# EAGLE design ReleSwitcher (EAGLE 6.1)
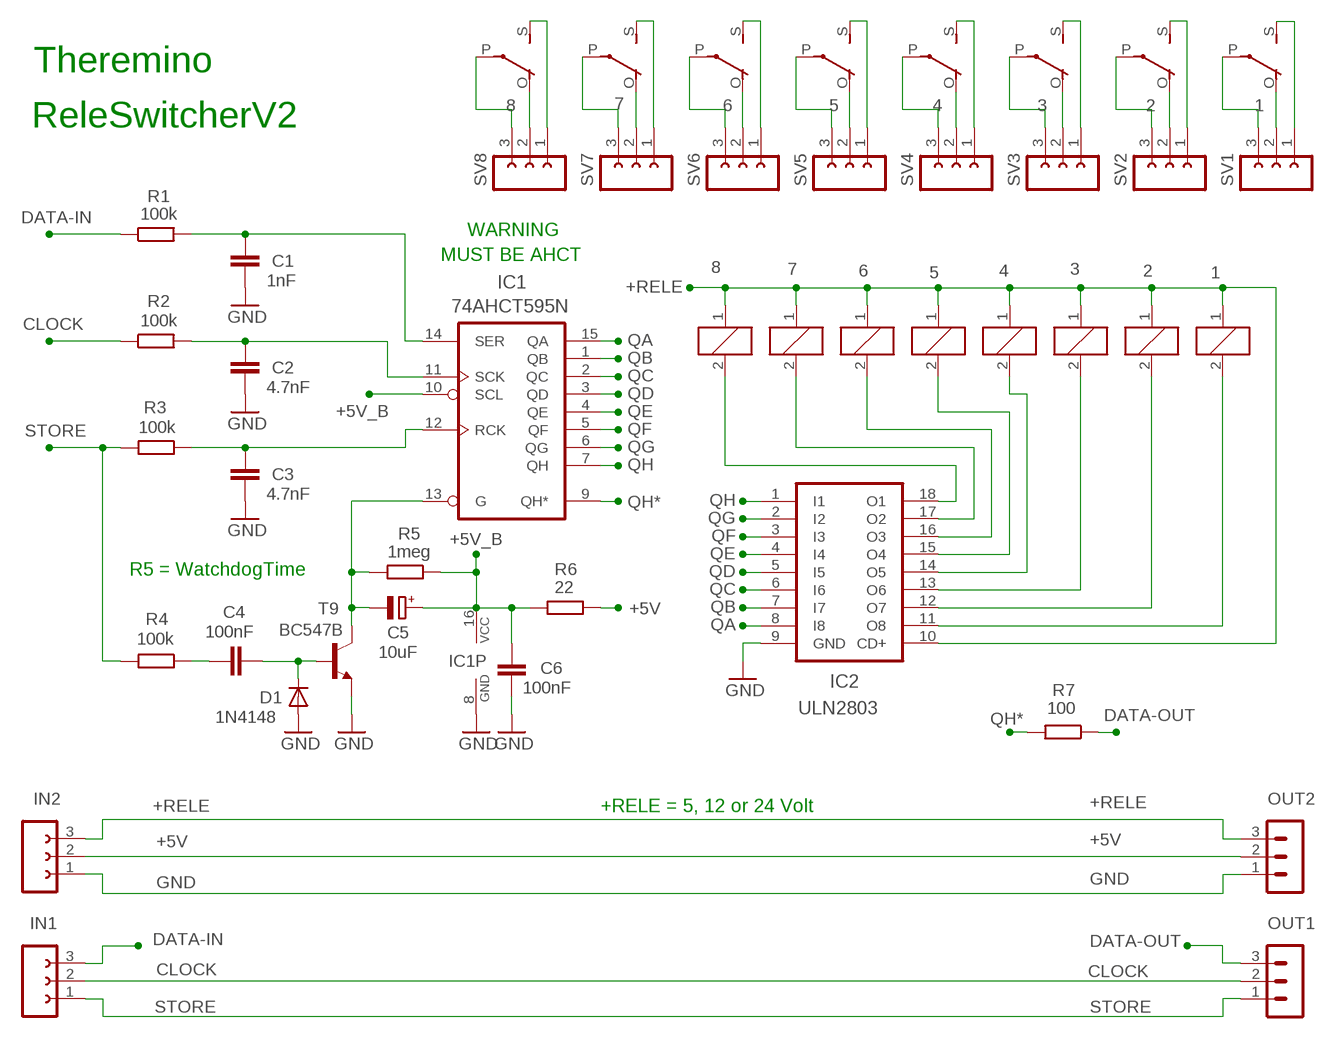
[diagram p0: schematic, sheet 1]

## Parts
1  E3206S  [E3206S]
2  E3206S  [E3206S]
3  E3206S  [E3206S]
4  E3206S  [E3206S]
5  E3206S  [E3206S]
6  E3206S  [E3206S]
7  E3206S  [E3206S]
8  E3206S  [E3206S]
C1  1nF  C-EU025-024X044  [C025-024X044]
C2  4.7nF  C-EU025-024X044  [C025-024X044]
C3  4.7nF  C-EU025-024X044  [C025-024X044]
C4  100nF  C-EU025-024X044  [C025-024X044]
C5  10uF  CPOL-EUE15-5AXIAL  [E15-5]
C6  100nF  C-EU025-024X044  [C025-024X044]
D1  1N4148  DIODE-D-5  [D-5]
IC1  74AHCT595N  74HCT595N  [DIL16]
IC2  ULN2803  ULN2803A  [DIL18]
IN1  FE03-1"  [FE03-1]
IN2  FE03-1"  [FE03-1]
OUT1  MA03-1N  [MA03-1]
OUT2  MA03-1N  [MA03-1]
R1  100k  R-EU_0207/10  [0207/10]
R2  100k  R-EU_0207/10  [0207/10]
R3  100k  R-EU_0207/10  [0207/10]
R4  100k  R-EU_0207/10  [0207/10]
R5  1meg  R-EU_0207/10  [0207/10]
R6  22  R-EU_0207/10  [0207/10]
R7  100  R-EU_0207/10  [0207/10]
SV1  CN-03"  [CN-03]
SV2  CN-03"  [CN-03]
SV3  CN-03"  [CN-03]
SV4  CN-03"  [CN-03]
SV5  CN-03"  [CN-03]
SV6  CN-03"  [CN-03]
SV7  CN-03"  [CN-03]
SV8  CN-03"  [CN-03]
T9  BC547B  -NPN-TO92-CBE  [TO92-CBE]

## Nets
+5V: IN2.2 OUT2.2 R6.1
+5V_B: C5.+ C6.1 IC1.10(SCL) IC1.16(VCC) R5.1 R6.2
+RELE: 1.1 2.1 3.1 4.1 5.1 6.1 7.1 8.1 IC2.10(CD+) IN2.3 OUT2.3
CLOCK: IN1.2 OUT1.2 R2.1
DATA-IN: IN1.3 R1.1
DATA-OUT: OUT1.3 R7.1
GND: C1.2 C2.2 C3.2 C6.2 D1.A IC1.8(GND) IC2.9(GND) IN2.1 OUT2.1 T9.E
N$1: 1.O(2:O) SV1.2
N$2: 1.P(2:P) SV1.3
N$3: C2.1 IC1.11(SCK) R2.2
N$4: 1.S(2:S) SV1.1
N$5: 2.S(2:S) SV2.1
N$6: 2.O(2:O) SV2.2
N$7: 3.2 IC2.13(O6)
N$8: 2.P(2:P) SV2.3
N$9: 3.S(2:S) SV3.1
N$10: 5.2 IC2.15(O4)
N$11: 6.2 IC2.16(O3)
N$12: 7.2 IC2.17(O2)
N$13: 8.2 IC2.18(O1)
N$14: 3.O(2:O) SV3.2
N$15: 3.P(2:P) SV3.3
N$16: C3.1 IC1.12(RCK) R3.1
N$17: C1.1 IC1.14(SER) R1.2
N$18: 4.S(2:S) SV4.1
N$19: 4.O(2:O) SV4.2
N$20: 4.P(2:P) SV4.3
N$21: 5.S(2:S) SV5.1
N$22: 5.O(2:O) SV5.2
N$23: 5.P(2:P) SV5.3
N$24: 6.S(2:S) SV6.1
N$25: 6.O(2:O) SV6.2
N$26: 6.P(2:P) SV6.3
N$27: 1.2 IC2.11(O8)
N$28: 2.2 IC2.12(O7)
N$29: 7.S(2:S) SV7.1
N$30: 4.2 IC2.14(O5)
N$31: 7.O(2:O) SV7.2
N$32: 7.P(2:P) SV7.3
N$33: 8.S(2:S) SV8.1
N$34: 8.O(2:O) SV8.2
N$35: 8.P(2:P) SV8.3
N$36: C4.1 R4.1
N$37: C5.- IC1.13(G) R5.2 T9.C
N$39: C4.2 D1.C T9.B
QA: IC1.15(QA) IC2.8(I8)
QB: IC1.1(QB) IC2.7(I7)
QC: IC1.2(QC) IC2.6(I6)
QD: IC1.3(QD) IC2.5(I5)
QE: IC1.4(QE) IC2.4(I4)
QF: IC1.5(QF) IC2.3(I3)
QG: IC1.6(QG) IC2.2(I2)
QH: IC1.7(QH) IC2.1(I1)
QH*: IC1.9(QH*) R7.2
STORE: IN1.1 OUT1.1 R3.2 R4.2

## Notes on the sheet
- Theremino
- ReleSwitcherV2
- WARNING
- MUST BE AHCT
- R5 = WatchdogTime
- +RELE = 5, 12 or 24 Volt

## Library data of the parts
1-8 = relay:E3206S: RELAY 1 x switch, Eichhoff/distributor Schukat
C1-C4 C6 = 00-LIVIO:C-EU: CAPACITOR, European symbol
C5 = 00-LIVIO:CPOL-EU: POLARIZED CAPACITOR, European symbol
D1 = 00-LIVIO:DIODE-: DIODE
IC1 = 74xx-eu:74*595: 8-bit SHIFT REGISTER, output latch
IC2 = uln-udn:ULN2803A: DRIVER ARRAY
IN1 IN2 = 02-con-lsta-F:FE03-1: FEMALE HEADER
OUT1 OUT2 = 03-con-lstb-M:MA03-1: PIN HEADER
R1-R7 = 00-LIVIO:R-EU_: RESISTOR, European symbol
SV1-SV8 = 01-Connettori_Vite_2.54:CN-03: Screw connector - Green - Spacing 2.54
T9 = 00-LIVIO:*-NPN-: NPN Transistror

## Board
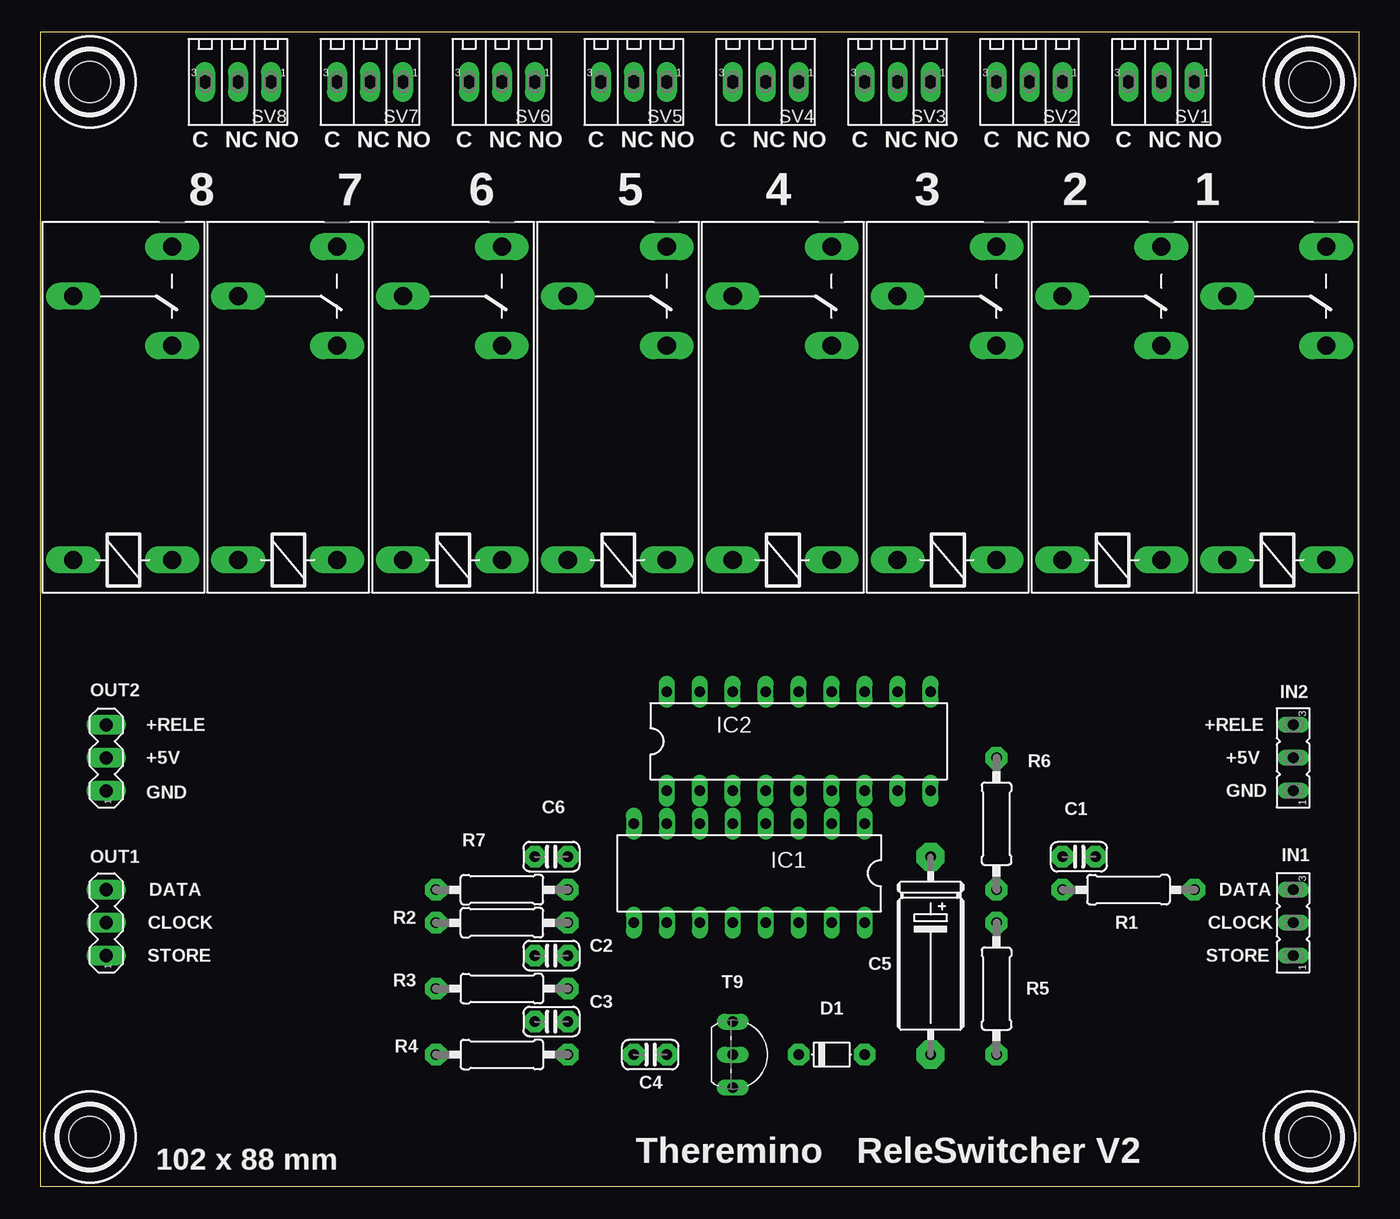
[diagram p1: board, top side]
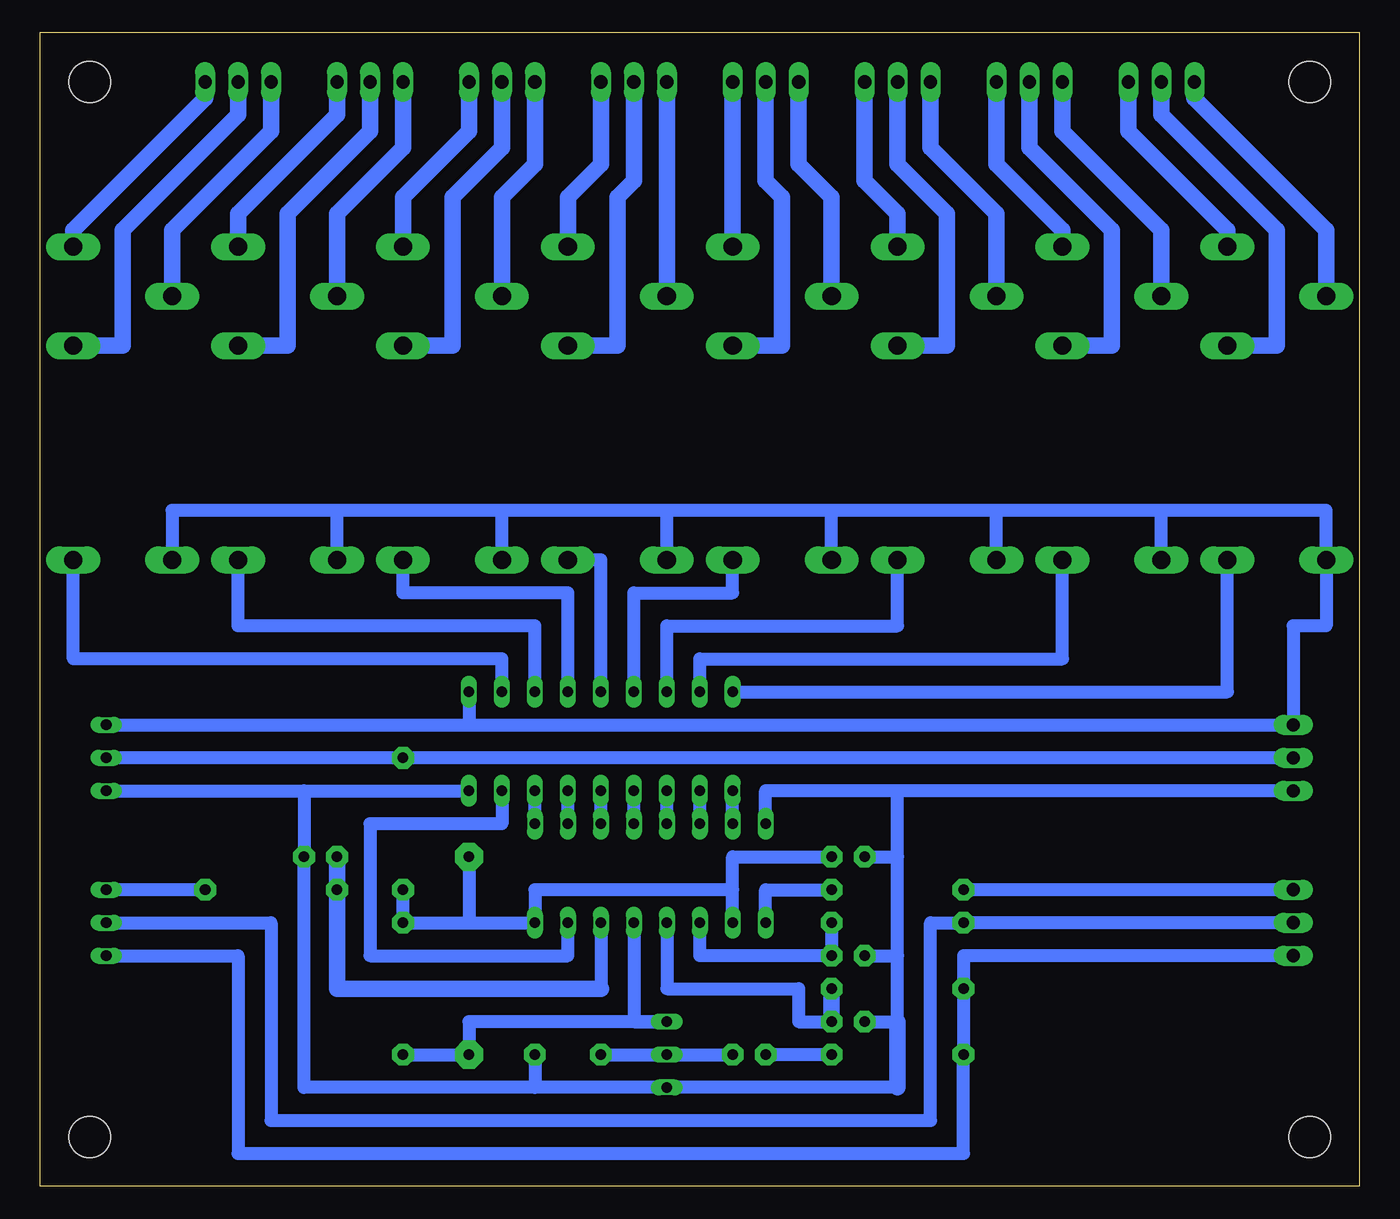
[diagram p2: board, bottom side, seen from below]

Size 101.6 x 88.9 mm. Coordinates in mm from the lower left corner, seen from the top.
Outline: 101.6,88.9 0,88.9 0,0 101.6,0 101.6,88.9
Copper layers (1*16): Top 0.035mm / dielectric 1.5mm / Bottom 0.035mm
Design rules: minimum track width 10mil, minimum drill 31mil, track to track 31mil, track to pad 31mil, pad to pad 31mil, via to via 31mil, smd to smd 31mil, copper to edge 31mil, drill to drill 8mil, minimum pad ring 5mil, minimum via ring 8mil, stop-mask expansion 4mil, vias tented up to drill 0mil, thermal gap 47mil
Holes 3.2 mm at 97.79,85.09 3.81,85.09 3.81,3.81 97.79,3.81

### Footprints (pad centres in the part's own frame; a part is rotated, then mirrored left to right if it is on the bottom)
E3206S = drill 1.397 long: 1 -3.175,3.81; 2 -3.175,-3.81; O 13.335,-3.81; P 17.145,3.81; S 20.955,-3.81
C025-024X044 = drill 0.813 pad 1.676 octagon: 1 -1.27,0; 2 1.27,0
E15-5 = drill 0.813 pad 2.159 octagon: + -7.62,0; - 7.62,0
D-5 = drill 0.813 pad 1.676 octagon: A 2.54,0; C -2.54,0
DIL16 = drill 0.813 long: 1 -8.89,-3.81; 2 -6.35,-3.81; 3 -3.81,-3.81; 4 -1.27,-3.81; 5 1.27,-3.81; 6 3.81,-3.81; 7 6.35,-3.81; 8 8.89,-3.81; 9 8.89,3.81; 10 6.35,3.81; 11 3.81,3.81; 12 1.27,3.81; 13 -1.27,3.81; 14 -3.81,3.81; 15 -6.35,3.81; 16 -8.89,3.81
DIL18 = drill 0.813 long: 1 -10.16,-3.81; 2 -7.62,-3.81; 3 -5.08,-3.81; 4 -2.54,-3.81; 5 0,-3.81; 6 2.54,-3.81; 7 5.08,-3.81; 8 7.62,-3.81; 9 10.16,-3.81; 10 10.16,3.81; 11 7.62,3.81; 12 5.08,3.81; 13 2.54,3.81; 14 0,3.81; 15 -2.54,3.81; 16 -5.08,3.81; 17 -7.62,3.81; 18 -10.16,3.81
FE03-1 = drill 0.813 long: 1 -2.54,0; 2 0,0; 3 2.54,0
MA03-1 = drill 1.016 long: 1 -2.54,0; 2 0,0; 3 2.54,0
0207/10 = drill 0.813 pad 1.676 octagon: 1 -5.08,0; 2 5.08,0
CN-03 = drill 1.016 pad 1.422 long: 1 -2.54,0; 2 0,0; 3 2.54,0
TO92-CBE = drill 0.813 long: B 0,0; C -2.54,0; E 2.54,0

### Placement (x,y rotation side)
1  95.25,51.43 90 top
2  82.55,51.43 90 top
3  69.85,51.43 90 top
4  57.15,51.43 90 top
5  44.45,51.43 90 top
6  31.75,51.43 90 top
7  19.05,51.43 90 top
8  6.35,51.43 90 top
C1  80.01,25.4 0 top
C2  39.37,17.78 180 top
C3  39.37,12.7 180 top
C4  46.99,10.16 0 top
C5  68.58,17.78 270 top
C6  39.37,25.4 180 top
D1  60.96,10.16 0 top
IC1  54.61,24.13 180 top
IC2  58.42,34.29 0 top
IN1  96.52,20.32 90 top
IN2  96.52,33.02 90 top
OUT1  5.08,20.32 90 top
OUT2  5.08,33.02 90 top
R1  83.82,22.86 180 top
R2  35.56,20.32 0 top
R3  35.56,15.24 180 top
R4  35.56,10.16 180 top
R5  73.66,15.24 270 top
R6  73.66,27.94 270 top
R7  35.56,22.86 0 top
SV1  86.36,85.09 180 top
SV2  76.2,85.09 180 top
SV3  66.04,85.09 180 top
SV4  55.88,85.09 180 top
SV5  45.72,85.09 180 top
SV6  35.56,85.09 180 top
SV7  25.4,85.09 180 top
SV8  15.24,85.09 180 top
T9  53.34,10.16 270 top

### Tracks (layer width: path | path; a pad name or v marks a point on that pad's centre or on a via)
+5V
  Bottom 1.016: IN2.2 R6.1 OUT2.2
+5V_B
  Bottom 1.016: 68.58,20.32 R5.1 R6.2 | C5.+ 68.58,20.32 | 68.58,20.32 IC1.16 63.5,22.86 48.26,22.86 IC1.10 48.26,25.4 C6.1
+RELE
  Bottom 1.016: 15.24,52.07 2.54,52.07 8.1 2.54,43.18 5.08,43.18 OUT2.3 68.58,35.56 | 15.24,52.07 27.94,52.07 | 27.94,52.07 40.64,52.07 | 40.64,52.07 53.34,52.07 | 53.34,52.07 66.04,52.07 | 66.04,52.07 78.74,52.07 | 78.74,52.07 91.44,52.07 1.1 | 7.1 15.24,52.07 | 6.1 27.94,52.07 | 5.1 40.64,52.07 | 4.1 53.34,52.07 | 3.1 66.04,52.07 | 2.1 78.74,52.07 | IC2.10 68.58,35.56 | IN2.3 68.58,35.56
CLOCK
  Bottom 1.016: OUT1.2 R2.1 33.02,20.32 33.02,5.08 83.82,5.08 83.82,20.32 IN1.2
DATA-IN
  Bottom 1.016: R1.1 IN1.3
DATA-OUT
  Bottom 1.016: OUT1.3 R7.1
GND
  Bottom 1.016: OUT2.1 35.56,30.48 | 35.56,30.48 45.72,30.48 IC1.8 | 81.28,30.48 IC2.9 | 35.56,7.62 T9.E 63.5,7.62 | 63.5,7.62 81.28,7.62 C1.2 81.28,30.48 | IN2.1 81.28,30.48 | 35.56,17.78 35.56,12.7 C3.2 | 35.56,17.78 35.56,25.4 | 35.56,25.4 35.56,30.48 | C2.2 35.56,17.78 | D1.A 63.5,7.62 | C6.2 35.56,25.4
  Bottom 1.27: 35.56,7.62 35.56,12.7
N$1
  Bottom 1.27: 1.O 95.25,64.77 95.25,73.66 86.36,82.55 SV1.2
N$2
  Bottom 1.27: 1.P 91.44,73.66 83.82,81.28 SV1.3
N$3
  Bottom 1.016: R2.2 C2.1 50.8,17.78 IC1.11
N$4
  Bottom 1.27: SV1.1 88.9,83.82 99.06,73.66 1.S
N$5
  Bottom 1.27: 2.S 86.36,74.93 78.74,82.55 SV2.1
N$6
  Bottom 1.27: 2.O 82.55,64.77 82.55,74.93 76.2,81.28 SV2.2
N$7
  Bottom 1.016: IC2.13 60.96,45.72 73.66,45.72 3.2
N$8
  Bottom 1.27: 2.P 78.74,74.93 73.66,80.01 SV2.3
N$9
  Bottom 1.27: 3.S 73.66,76.2 68.58,81.28 SV3.1
N$10
  Bottom 1.016: IC2.15 55.88,45.72 48.26,45.72 5.2
N$11
  Bottom 1.016: IC2.16 53.34,43.18 35.56,43.18 6.2
N$12
  Bottom 1.016: IC2.17 50.8,40.64 22.86,40.64 7.2
N$13
  Bottom 1.016: IC2.18 10.16,38.1 8.2
N$14
  Bottom 1.27: 3.O 69.85,64.77 69.85,76.2 66.04,80.01 SV3.2
N$15
  Bottom 1.27: 3.P 66.04,76.2 63.5,78.74 SV3.3
N$16
  Bottom 1.016: IC1.12 53.34,15.24 43.18,15.24 43.18,12.7 C3.1
  Bottom 1.27: C3.1 R3.1
N$17
  Bottom 1.016: IC1.14 58.42,15.24
  Bottom 1.27: 58.42,15.24 78.74,15.24 R1.2 C1.1
N$18
  Bottom 1.27: 4.S 60.96,76.2 58.42,78.74 SV4.1
N$19
  Bottom 1.27: 4.O 57.15,64.77 57.15,76.2 55.88,77.47 SV4.2
N$20
  Bottom 1.27: 4.P SV4.3
N$21
  Bottom 1.27: 5.S SV5.1
N$22
  Bottom 1.27: 5.O 44.45,64.77 44.45,76.2 45.72,77.47 SV5.2
N$23
  Bottom 1.27: 5.P 40.64,76.2 43.18,78.74 SV5.3
N$24
  Bottom 1.27: 6.S 35.56,74.93 38.1,77.47 SV6.1
N$25
  Bottom 1.27: 6.O 31.75,64.77 31.75,74.93 35.56,78.74 SV6.2
N$26
  Bottom 1.27: 6.P 27.94,74.93 33.02,80.01 SV6.3
N$27
  Bottom 1.016: IC2.11 66.04,40.64 99.06,40.64 1.2
N$28
  Bottom 1.016: IC2.12 63.5,43.18 86.36,43.18 2.2
N$29
  Bottom 1.27: 7.S 22.86,73.66 27.94,78.74 SV7.1
N$30
  Bottom 1.016: IC2.14 58.42,48.26 4.2
N$31
  Bottom 1.27: 7.O 19.05,64.77 19.05,73.66 25.4,80.01 SV7.2
N$32
  Bottom 1.27: 7.P 15.24,73.66 22.86,81.28 SV7.3
N$33
  Bottom 1.27: 8.S 10.16,73.66 17.78,81.28 SV8.1
N$34
  Bottom 1.27: 8.O 6.35,64.77 6.35,73.66 15.24,82.55 SV8.2
N$35
  Bottom 1.27: 8.P 2.54,73.66 12.7,83.82 SV8.3
N$36
  Bottom 1.016: R4.1 C4.1
N$37
  Bottom 1.016: IC1.13 55.88,12.7 T9.C 68.58,12.7 C5.- R5.2
N$39
  Bottom 1.016: D1.C T9.B C4.2
QA
  Bottom 1.016: IC2.8 66.04,27.94 76.2,27.94 76.2,17.78 60.96,17.78 IC1.15
QB
  Bottom 1.016: IC1.1 IC2.7
QC
  Bottom 1.016: IC1.2 IC2.6
QD
  Bottom 1.016: IC1.3 IC2.5
QE
  Bottom 1.016: IC1.4 IC2.4
QF
  Bottom 1.016: IC1.5 IC2.3
QG
  Bottom 1.016: IC1.6 IC2.2
QH
  Bottom 1.016: IC1.7 IC2.1
QH*
  Bottom 1.016: IC1.9 45.72,22.86 R7.2
STORE
  Bottom 1.016: OUT1.1 30.48,17.78 R3.2 R4.2 30.48,2.54 86.36,2.54 86.36,17.78 IN1.1

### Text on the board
tNames: C | NC | NO | C | NC | NO | C | NC | NO | C | NC | NO | C | NC | NO | C | NC | NO | C | NC | NO | C | NC | NO | +RELE | +RELE | +5V | +5V | GND | GND | DATA | DATA | CLOCK | CLOCK | STORE | STORE | Theremino | ReleSwitcher V2 | 102 x 88 mm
